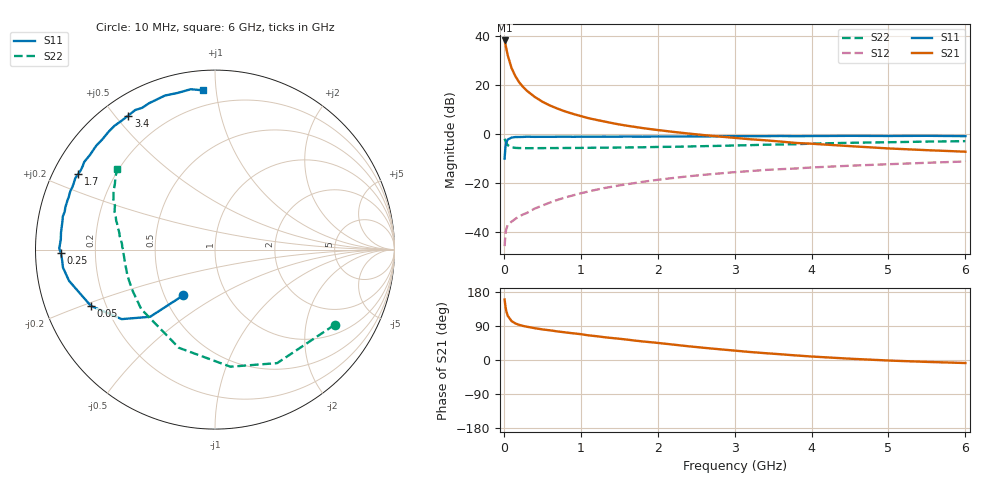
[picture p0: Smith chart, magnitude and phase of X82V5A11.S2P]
! SIEMENS Small Signal Semiconductors
! BFP136W
! Si NPN RF Bipolar Junction Transistor in SOT343
! VCE = 2.5 V  IC = 110 mA
! Common Emitter S-Parameters:  September  1994
# GHz  S  MA  R  50
!  f  S11  S21  S12  S22
! GHz  MAG  ANG  MAG  ANG  MAG  ANG  MAG  ANG
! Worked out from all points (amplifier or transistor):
!   40 points, 10 MHz to 6 GHz, reference 50 ohm
!   highest |S21| = 38.0 dB at 10 MHz (marker M1)
!   |S21| within 3 dB of that: start of sweep to 30.16 MHz
!   unconditionally stable (mu >= 1): 468.1 MHz to 2.856 GHz
!   at 200 MHz: K = 0.72, MSG = 27.3 dB, |S12| = -33.7 dB
!   at 1.5 GHz: K = 1.10, MAG = 10.5 dB, |S12| = -21.1 dB
!   at 6 GHz: K = 0.98, MSG = 2.0 dB, |S12| = -11.3 dB
!   S11 on the Smith chart (normalised r, x): 10 MHz: 0.62, -0.35; 50 MHz: 0.14, -0.21; 250 MHz: 0.08, -0.01; 1.7 GHz: 0.07, +0.26; 3.4 GHz: 0.08, +0.54; 6 GHz: 0.11, +0.92
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0.01  0.3109 -124.8  79.28 159.5  0.0051 68.1  0.7871 -32.2
0.02  0.5204 -134.0  67.34 142.6  0.0086 54.9  0.721 -61.3
0.03  0.6482 -143.3  56.27 130.7  0.0112 47.1  0.6581 -82.5
0.05  0.7593 -155.6  39.72 116.9  0.0137 37.1  0.583 -110.2
0.1  0.8315 -167.9  21.78 102.7  0.0161 36.8  0.5281 -141.1
0.15  0.853 -173.3  14.8 96.5  0.0184 40.9  0.5132 -153.5
0.2  0.8541 -176.3  11.09 92.7  0.0206 43.5  0.5091 -160.2
0.25  0.8592 -178.8  8.948 89.9  0.0226 46.7  0.5081 -164.5
0.3  0.8677 179.6  7.476 87.8  0.0243 50.0  0.5064 -167.4
0.4  0.8609 176.1  5.631 84.0  0.0297 54.6  0.5068 -171.2
0.5  0.8633 173.7  4.487 80.8  0.0343 57.3  0.5075 -173.8
0.6  0.8632 171.8  3.746 78.3  0.0395 59.7  0.5082 -175.5
0.7  0.8647 169.2  3.227 75.3  0.0449 61.1  0.5096 -176.8
0.9  0.8636 165.8  2.527 70.4  0.0553 62.4  0.5111 -179.4
1.1  0.8663 161.5  2.069 65.0  0.0663 62.5  0.5148 179.0
1.7  0.8711 151.0  1.376 51.3  0.0984 60.0  0.526 174.1
2.2  0.8737 142.7  1.088 40.7  0.1249 56.0  0.54 170.4
3.2  0.8867 125.9  0.77 21.1  0.1727 46.1  0.583 161.6
3.4  0.8896 122.9  0.732 18.0  0.1823 43.8  0.5959 159.8
4.5  0.9024 108.0  0.557 3.4  0.2222 33.5  0.6512 150.2
5.5  0.9037 98.6  0.461 -5.0  0.255 25.5  0.6891 143.5
6  0.8901 94.4  0.429 -8.0  0.2712 21.1  0.704 140.5
